|   stm32f765_767_777_bga176 IBIS Model
[IBIS ver]   4.2
[File name]  stm32f765_767_777_bga176.ibs
[File Rev]   1.0
[Date]   24-06-2015
[Source] Data Created at STMicroelectronics
[Notes]   File originated from ELDO simulations.
[Disclaimer]  This information is for modeling purpose only and is
   not guaranted. The information is subject to change without
   notice.
[Copyright] Copyright 2016 STMicroelectronics Inc.
[Component] stm32f765_767_777_bga176
[Manufacturer] STMicroelectronics
[Package]
| variable   typ   min   max
R_pkg   0.0   NA   NA
L_pkg   0.0H   NA   NA
C_pkg   0.0F   NA   NA
[Pin]   signal_name   model_name   R_pin   L_pin   C_pin
A1 PE3 io8p_arsudq_ft
A10 PB3 io8p_arsudq_ft
A11 PD7 io8p_arsudq_ft
A12 PC12 io8p_arsudq_ft
A13 PA15 io8p_arsudq_ft
A14 PA14 io8p_arsudq_ft
A15 PA13 io8p_arsudq_ft
A2 PE2 io8p_arsudq_ft
A3 PE1 io8p_arsudq_ft
A4 PE0 io8p_arsudq_ft
A5 PB8 io8p_arsudq_i2cin_ft
A6 PB5 io8p_ar3wsudq_ft
A7 PG14 io8p_arsudq_ft
A8 PG13 io8p_arsudq_ft
A9 PB4 io8p_arsudq_ft
B1 PE4 io8p_arsudq_ft
B10 PG10 io8p_arsudq_ft
B11 PD6 io8p_arsudq_ft
B12 PD0 io8p_arsudq_ft
B13 PC11 io8p_arsudq_ft
B14 PC10 io8p_arsudq_ft
B15 PA12 io8usb_lsfs_otg_ft
B2 PE5 io8p_arsudq_ft
B3 PE6 io8p_arsudq_ft
B4 PB9 io8p_arsudq_i2cin_ft
B5 PB7 io8p_arsudq_i2cin_ft
B6 PB6 io8p_arsudq_i2cin_ft
B7 PG15 io8p_arsudq_ft
B8 PG12 io8p_arsudq_ft
B9 PG11 io8p_arsudq_ft
C1 VBAT POWER
C10 PG9 io8p_arsudq_ft
C11 PD5 io8p_arsudq_ft
C12 PD1 io8p_arsudq_ft
C13 PI3 io8p_arsudq_ft
C14 PI2 io8p_arsudq_ft
C15 PA11 io8usb_lsfs_otg_ft
C2 PI7 io8p_arsudq_ft
C3 PI6 io8p_arsudq_ft
C4 PI5 io8p_arsudq_ft
C5 VDD POWER
C6 PDR_ON NC
C7 VDD POWER
C8 VDDSDMMC POWER
C9 VDD POWER
D1 PC13 io8p_arwsudq_ft_v33
D10 PD4 io8p_arsudq_ft
D11 PD3 io8p_arsudq_ft
D12 PD2 io8p_arsudq_ft
D13 PH15 io8p_arsudq_ft
D14 PI1 io8p_arsudq_ft
D15 PA10 io8usb_id_otg_ft
D2 PI8 io8p_arsudq_ft_v33
D3 PI9 io8p_arsudq_ft
D4 PI4 io8p_arsudq_ft
D5 VSS GND
D6 BOOT0 GND
D7 VSS GND
D8 VSS GND
D9 VSS GND
E1 PC14-OSC32_IN io8p_arwsudq_ft_v33
E12 PH13 io8p_arsudq_ft
E13 PH14 io8p_arsudq_ft
E14 PI0 io8p_arsudq_ft
E15 PA9 io8usb_vbus_otg_ft
E2 PF0 io8p_arsudq_i2cin_ft
E3 PI10 io8p_arsudq_ft
E4 PI11 io8p_arsudq_ft_v33
F1 PC15-OSC32_OUT io8p_arsudq_ft
F12 VSS GND
F13 VCAP_2 POWER
F14 PC9 io8p_arsudq_i2cin_ft
F15 PA8 io8p_arsudq_i2cin_ft
F2 VSS GND
F3 VDD POWER
F4 PH2 io8p_arsudq_ft
F6 VSS GND
F7 VSS GND
F8 VSS GND
F9 VSS GND
F10 VSS GND
G1 PH0-OSC_IN io8p_arsudq_ft
G12 VSS GND
G13 VDD POWER
G14 PC8 io8p_arsudq_ft
G15 PC7 io8p_arsudq_ft
G2 VSS GND
G3 VDD POWER
G4 PH3 io8p_arsudq_ft
G6 VSS GND
G7 VSS GND
G8 VSS GND
G9 VSS GND
G10 VSS GND
H1 PH1-OSC_OUT io8p_arsudq_ft
H12 VSS GND
H13 VDDUSB POWER
H14 PG8 io8p_arsudq_ft
H15 PC6 io8p_arsudq_ft
H2 PF2 io8p_arsudq_ft
H3 PF1 io8p_arsudq_i2cin_ft
H4 PH4 io8p_arsudq_i2cin_ft
H6 VSS GND
H7 VSS GND
H8 VSS GND
H9 VSS GND
H10 VSS GND
J1 NRST ioreset_ft_v33
J12 VDD POWER
J13 VDD POWER
J14 PG7 io8p_arsudq_ft
J15 PG6 io8p_arsudq_ft
J2 PF3 io8p_arwsudq_ft
J3 PF4 io8p_arwsudq_ft
J4 PH5 io8p_arsudq_i2cin_ft
J6 VSS GND
J7 VSS GND
J8 VSS GND
J9 VSS GND
J10 VSS GND
K1 PF7 io8p_arwsudq_ft
K12 PH12 io8p_arsudq_i2cin_ft
K13 PG5 io8p_arsudq_ft
K14 PG4 io8p_arsudq_ft
K15 PG3 io8p_arsudq_ft
K2 PF6 io8p_arwsudq_ft
K3 PF5 io8p_arwsudq_ft
K4 VDD POWER
K6 VSS GND
K7 VSS GND
K8 VSS GND
K9 VSS GND
K10 VSS GND
L1 PF10 io8p_arwsudq_ft
L12 PH11 io8p_arsudq_i2cin_ft
L13 PH10 io8p_arsudq_ft
L14 PD15 io8p_arsudq_ft
L15 PG2 io8p_arsudq_ft
L2 PF9 io8p_arwsudq_ft
L3 PF8 io8p_arwsudq_ft
L4 BYPASS_REG NC
M1 VSSA GND
M10 VCAP_1 POWER
M11 PH6 io8p_arsudq_ft
M12 PH8 io8p_arsudq_i2cin_ft
M13 PH9 io8p_arsudq_ft
M14 PD14 io8p_arsudq_ft
M15 PD13 io8p_arsudq_i2cin_ft
M2 PC0 io8p_ar3wsudq_ft
M3 PC1 io8p_ar3wsudq_ft_v33
M4 PC2 io8p_ar3wsudq_ft
M5 PC3 io8p_ar3wsudq_ft
M6 PB2 io8p_ar3wsudq_ft
M7 PG1 io8p_arsudq_ft
M8 VSS GND
M9 VSS GND
N1 VREF- GND
N10 VDD POWER
N11 PE13 io8p_arsudq_ft
N12 PH7 io8p_arsudq_i2cin_ft
N13 PD12 io8p_arsudq_i2cin_ft
N14 PD11 io8p_arsudq_ft
N15 PD10 io8p_arsudq_ft
N2 PA1 io8p_ar3wsudq_ft
N3 PA0-WKUP io8p_ar3wsudq_ft_v33
N4 PA4 io8p_ar3wsudq_ft
N5 PC4 io8p_ar3wsudq_ft
N6 PF13 io8p_arsudq_ft
N7 PG0 io8p_arsudq_ft
N8 VDD POWER
N9 VDD POWER
P1 VREF+ POWER
P10 PE11 io8p_arsudq_ft
P11 PE14 io8p_arsudq_ft
P12 PB12 io8usb_id_otg_ft
P13 PB13 io8usb_vbus_otg_ft
P14 PD9 io8p_arsudq_ft
P15 PD8 io8p_arsudq_ft
P2 PA2 io8p_ar3wsudq_ft_v33
P3 PA6 io8p_ar3wsudq_ft
P4 PA5 io8p_ar3wsudq_ft
P5 PC5 io8p_ar3wsudq_ft
P6 PF12 io8p_arsudq_ft
P7 PF15 io8p_arsudq_i2cin_ft
P8 PE8 io8p_arsudq_ft
P9 PE9 io8p_arsudq_ft
R1 VDDA POWER
R10 PE12 io8p_arsudq_ft
R11 PE15 io8p_ar3wsudq_ft
R12 PB10 io8p_arsudq_i2cin_ft
R13 PB11 io8p_arsudq_i2cin_ft
R14 PB14 io8usb_lsfs_otg_ft
R15 PB15 io8usb_lsfs_otg_ft
R2 PA3 io8p_ar3wsudq_ft
R3 PA7 io8p_ar3wsudq_ft
R4 PB1 io8p_ar3wsudq_ft
R5 PB0 io8p_ar3wsudq_ft
R6 PF11 io8p_arsudq_ft
R7 PF14 io8p_arsudq_i2cin_ft
R8 PE7 io8p_arsudq_ft
R9 PE10 io8p_arsudq_ft
[Diff Pin]   inv_pin   vdiff   tdelay_typ  tdelay_min  tdelay_max
C15   B15   200mV   NA   NA   NA
R14   R15   200mV   NA   NA   NA
[Model Selector] io8p_ar3wsudq_ft
io8p00_ar3wsudq_ft_pd_lv  "SPEED00 1P8V, PD=40kOhm"
io8p00_ar3wsudq_ft_pu_lv  "SPEED00 1P8V, PU=40kOhm"
io8p00_ar3wsudq_ft_lv  "SPEED00 1P8V"
io8p01_ar3wsudq_ft_pd_lv  "SPEED01 1P8V, PD=40kOhm"
io8p01_ar3wsudq_ft_pu_lv  "SPEED01 1P8V, PU=40kOhm"
io8p01_ar3wsudq_ft_lv  "SPEED01 1P8V"
io8p10_ar3wsudq_ft_pd_lv  "SPEED10 1P8V, PD=40kOhm"
io8p10_ar3wsudq_ft_pu_lv  "SPEED10 1P8V, PU=40kOhm"
io8p10_ar3wsudq_ft_lv  "SPEED10 1P8V"
io8p11_ar3wsudq_ft_pd_lv  "SPEED11 1P8V, PD=40kOhm"
io8p11_ar3wsudq_ft_pu_lv  "SPEED11 1P8V, PU=40kOhm"
io8p11_ar3wsudq_ft_lv  "SPEED11 1P8V"
io8p00_ar3wsudq_ft_pd  "SPEED00, PD=40kOhm"
io8p00_ar3wsudq_ft_pu  "SPEED00, PU=40kOhm"
io8p00_ar3wsudq_ft  "SPEED00"
io8p01_ar3wsudq_ft_pd  "SPEED01, PD=40kOhm"
io8p01_ar3wsudq_ft_pu  "SPEED01, PU=40kOhm"
io8p01_ar3wsudq_ft  "SPEED01"
io8p10_ar3wsudq_ft_pd  "SPEED10, PD=40kOhm"
io8p10_ar3wsudq_ft_pu  "SPEED10, PU=40kOhm"
io8p10_ar3wsudq_ft  "SPEED10"
io8p11_ar3wsudq_ft_pd  "SPEED11, PD=40kOhm"
io8p11_ar3wsudq_ft_pu  "SPEED11, PU=40kOhm"
io8p11_ar3wsudq_ft  "SPEED11"
[Model Selector] io8p_ar3wsudq_ft_v33
io8p00_ar3wsudq_ft_v33_pd_lv  "SPEED00 1P8V, PD=40kOhm"
io8p00_ar3wsudq_ft_v33_pu_lv  "SPEED00 1P8V, PU=40kOhm"
io8p00_ar3wsudq_ft_v33_lv  "SPEED00 1P8V"
io8p01_ar3wsudq_ft_v33_pd_lv  "SPEED01 1P8V, PD=40kOhm"
io8p01_ar3wsudq_ft_v33_pu_lv  "SPEED01 1P8V, PU=40kOhm"
io8p01_ar3wsudq_ft_v33_lv  "SPEED01 1P8V"
io8p10_ar3wsudq_ft_v33_pd_lv  "SPEED10 1P8V, PD=40kOhm"
io8p10_ar3wsudq_ft_v33_pu_lv  "SPEED10 1P8V, PU=40kOhm"
io8p10_ar3wsudq_ft_v33_lv  "SPEED10 1P8V"
io8p11_ar3wsudq_ft_v33_pd_lv  "SPEED11 1P8V, PD=40kOhm"
io8p11_ar3wsudq_ft_v33_pu_lv  "SPEED11 1P8V, PU=40kOhm"
io8p11_ar3wsudq_ft_v33_lv  "SPEED11 1P8V"
io8p00_ar3wsudq_ft_v33_pd  "SPEED00, PD=40kOhm"
io8p00_ar3wsudq_ft_v33_pu  "SPEED00, PU=40kOhm"
io8p00_ar3wsudq_ft_v33  "SPEED00"
io8p01_ar3wsudq_ft_v33_pd  "SPEED01, PD=40kOhm"
io8p01_ar3wsudq_ft_v33_pu  "SPEED01, PU=40kOhm"
io8p01_ar3wsudq_ft_v33  "SPEED01"
io8p10_ar3wsudq_ft_v33_pd  "SPEED10, PD=40kOhm"
io8p10_ar3wsudq_ft_v33_pu  "SPEED10, PU=40kOhm"
io8p10_ar3wsudq_ft_v33  "SPEED10"
io8p11_ar3wsudq_ft_v33_pd  "SPEED11, PD=40kOhm"
io8p11_ar3wsudq_ft_v33_pu  "SPEED11, PU=40kOhm"
io8p11_ar3wsudq_ft_v33  "SPEED11"
[Model Selector] io8p_arsudq_ft
io8p00_arsudq_ft_pd_lv  "SPEED00 1P8V, PD=40kOhm"
io8p00_arsudq_ft_pu_lv  "SPEED00 1P8V, PU=40kOhm"
io8p00_arsudq_ft_lv  "SPEED00 1P8V"
io8p01_arsudq_ft_pd_lv  "SPEED01 1P8V, PD=40kOhm"
io8p01_arsudq_ft_pu_lv  "SPEED01 1P8V, PU=40kOhm"
io8p01_arsudq_ft_lv  "SPEED01 1P8V"
io8p10_arsudq_ft_pd_lv  "SPEED10 1P8V, PD=40kOhm"
io8p10_arsudq_ft_pu_lv  "SPEED10 1P8V, PU=40kOhm"
io8p10_arsudq_ft_lv  "SPEED10 1P8V"
io8p11_arsudq_ft_pd_lv  "SPEED11 1P8V, PD=40kOhm"
io8p11_arsudq_ft_pu_lv  "SPEED11 1P8V, PU=40kOhm"
io8p11_arsudq_ft_lv  "SPEED11 1P8V"
io8p00_arsudq_ft_pd  "SPEED00, PD=40kOhm"
io8p00_arsudq_ft_pu  "SPEED00, PU=40kOhm"
io8p00_arsudq_ft  "SPEED00"
io8p01_arsudq_ft_pd  "SPEED01, PD=40kOhm"
io8p01_arsudq_ft_pu  "SPEED01, PU=40kOhm"
io8p01_arsudq_ft  "SPEED01"
io8p10_arsudq_ft_pd  "SPEED10, PD=40kOhm"
io8p10_arsudq_ft_pu  "SPEED10, PU=40kOhm"
io8p10_arsudq_ft  "SPEED10"
io8p11_arsudq_ft_pd  "SPEED11, PD=40kOhm"
io8p11_arsudq_ft_pu  "SPEED11, PU=40kOhm"
io8p11_arsudq_ft  "SPEED11"
[Model Selector] io8p_arsudq_i2cin_ft
io8p00_arsudq_i2cin_ft_pd_lv  "SPEED00 1P8V, PD=40kOhm"
io8p00_arsudq_i2cin_ft_pu_lv  "SPEED00 1P8V, PU=40kOhm"
io8p00_arsudq_i2cin_ft_lv  "SPEED00 1P8V"
io8p01_arsudq_i2cin_ft_pd_lv  "SPEED01 1P8V, PD=40kOhm"
io8p01_arsudq_i2cin_ft_pu_lv  "SPEED01 1P8V, PU=40kOhm"
io8p01_arsudq_i2cin_ft_lv  "SPEED01 1P8V"
io8p10_arsudq_i2cin_ft_pd_lv  "SPEED10 1P8V, PD=40kOhm"
io8p10_arsudq_i2cin_ft_pu_lv  "SPEED10 1P8V, PU=40kOhm"
io8p10_arsudq_i2cin_ft_lv  "SPEED10 1P8V"
io8p11_arsudq_i2cin_ft_pd_lv  "SPEED11 1P8V, PD=40kOhm"
io8p11_arsudq_i2cin_ft_pu_lv  "SPEED11 1P8V, PU=40kOhm"
io8p11_arsudq_i2cin_ft_lv  "SPEED11 1P8V"
io8p00_arsudq_i2cin_ft_pd  "SPEED00, PD=40kOhm"
io8p00_arsudq_i2cin_ft_pu  "SPEED00, PU=40kOhm"
io8p00_arsudq_i2cin_ft  "SPEED00"
io8p01_arsudq_i2cin_ft_pd  "SPEED01, PD=40kOhm"
io8p01_arsudq_i2cin_ft_pu  "SPEED01, PU=40kOhm"
io8p01_arsudq_i2cin_ft  "SPEED01"
io8p10_arsudq_i2cin_ft_pd  "SPEED10, PD=40kOhm"
io8p10_arsudq_i2cin_ft_pu  "SPEED10, PU=40kOhm"
io8p10_arsudq_i2cin_ft  "SPEED10"
io8p11_arsudq_i2cin_ft_pd  "SPEED11, PD=40kOhm"
io8p11_arsudq_i2cin_ft_pu  "SPEED11, PU=40kOhm"
io8p11_arsudq_i2cin_ft  "SPEED11"
[Model Selector] io8p_arwsudq_ft_v33
io8p00_arwsudq_ft_v33_pd_lv  "SPEED00 1P8V, PD=40kOhm"
io8p00_arwsudq_ft_v33_pu_lv  "SPEED00 1P8V, PU=40kOhm"
io8p00_arwsudq_ft_v33_lv  "SPEED00 1P8V"
io8p01_arwsudq_ft_v33_pd_lv  "SPEED01 1P8V, PD=40kOhm"
io8p01_arwsudq_ft_v33_pu_lv  "SPEED01 1P8V, PU=40kOhm"
io8p01_arwsudq_ft_v33_lv  "SPEED01 1P8V"
io8p10_arwsudq_ft_v33_pd_lv  "SPEED10 1P8V, PD=40kOhm"
io8p10_arwsudq_ft_v33_pu_lv  "SPEED10 1P8V, PU=40kOhm"
io8p10_arwsudq_ft_v33_lv  "SPEED10 1P8V"
io8p11_arwsudq_ft_v33_pd_lv  "SPEED11 1P8V, PD=40kOhm"
io8p11_arwsudq_ft_v33_pu_lv  "SPEED11 1P8V, PU=40kOhm"
io8p11_arwsudq_ft_v33_lv  "SPEED11 1P8V"
io8p00_arwsudq_ft_v33_pd  "SPEED00, PD=40kOhm"
io8p00_arwsudq_ft_v33_pu  "SPEED00, PU=40kOhm"
io8p00_arwsudq_ft_v33  "SPEED00"
io8p01_arwsudq_ft_v33_pd  "SPEED01, PD=40kOhm"
io8p01_arwsudq_ft_v33_pu  "SPEED01, PU=40kOhm"
io8p01_arwsudq_ft_v33  "SPEED01"
io8p10_arwsudq_ft_v33_pd  "SPEED10, PD=40kOhm"
io8p10_arwsudq_ft_v33_pu  "SPEED10, PU=40kOhm"
io8p10_arwsudq_ft_v33  "SPEED10"
io8p11_arwsudq_ft_v33_pd  "SPEED11, PD=40kOhm"
io8p11_arwsudq_ft_v33_pu  "SPEED11, PU=40kOhm"
io8p11_arwsudq_ft_v33  "SPEED11"
[Model Selector] io8usb_id_otg_ft
io8p00_id_otg_ft_pd_lv  "SPEED00 1P8V, PD=14kOhm"
io8p00_id_otg_ft_pu_lv  "SPEED00 1P8V, PU=14kOhm"
io8p00_id_otg_ft_lv  "SPEED00 1P8V"
io8p01_id_otg_ft_pd_lv  "SPEED01 1P8V, PD=14kOhm"
io8p01_id_otg_ft_pu_lv  "SPEED01 1P8V, PU=14kOhm"
io8p01_id_otg_ft_lv  "SPEED01 1P8V"
io8p10_id_otg_ft_pd_lv  "SPEED10 1P8V, PD=14kOhm"
io8p10_id_otg_ft_pu_lv  "SPEED10 1P8V, PU=14kOhm"
io8p10_id_otg_ft_lv  "SPEED10 1P8V"
io8p11_id_otg_ft_pd_lv  "SPEED11 1P8V, PD=14kOhm"
io8p11_id_otg_ft_pu_lv  "SPEED11 1P8V, PU=14kOhm"
io8p11_id_otg_ft_lv  "SPEED11 1P8V"
io8p00_id_otg_ft_pd  "SPEED00, PD=14kOhm"
io8p00_id_otg_ft_pu  "SPEED00, PU=14kOhm"
io8p00_id_otg_ft  "SPEED00"
io8p01_id_otg_ft_pd  "SPEED01, PD=14kOhm"
io8p01_id_otg_ft_pu  "SPEED01, PU=14kOhm"
io8p01_id_otg_ft  "SPEED01"
io8p10_id_otg_ft_pd  "SPEED10, PD=14kOhm"
io8p10_id_otg_ft_pu  "SPEED10, PU=14kOhm"
io8p10_id_otg_ft  "SPEED10"
io8p11_id_otg_ft_pd  "SPEED11, PD=14kOhm"
io8p11_id_otg_ft_pu  "SPEED11, PU=14kOhm"
io8p11_id_otg_ft  "SPEED11"
[Model Selector] io8usb_lsfs_otg_ft
io8usb_ls_otg_ft_dpdn_pd  "LS USB DP/DN IO + PD=20kOhm"
io8usb_ls_otg_ft_dpdn_pupu2  "LS USB DP/DN IO + PU/PU2=2.2kOhm"
io8usb_ls_otg_ft_dpdn_pu2  "LS USB DP/DN IO + PU2=1.2kOhm"
io8usb_ls_otg_ft_dpdn_pu  "LS USB DP/DN IO + PU=1.2kOhm"
io8usb_ls_otg_ft_dpdn  "LS USB DP/DN IO"
io8usb_fs_otg_ft_dpdn_pd  "HS USB DP/DN IO + PD=20kOhm"
io8usb_fs_otg_ft_dpdn_pupu2  "HS USB DP/DN IO + PU/PU2=2.2kOhm"
io8usb_fs_otg_ft_dpdn_pu2  "HS USB DP/DN IO + PU2=1.2kOhm"
io8usb_fs_otg_ft_dpdn_pu  "HS USB DP/DN IO + PU=1.2kOhm"
io8usb_fs_otg_ft_dpdn  "HS USB DP/DN IO"
io8p00_lsfs_otg_ft_pd_lv  "SPEED00 1P8V, PD=40kOhm"
io8p00_lsfs_otg_ft_pu_lv  "SPEED00 1P8V, PU=40kOhm"
io8p00_lsfs_otg_ft_lv  "SPEED00 1P8V"
io8p01_lsfs_otg_ft_pd_lv  "SPEED01 1P8V, PD=40kOhm"
io8p01_lsfs_otg_ft_pu_lv  "SPEED01 1P8V, PU=40kOhm"
io8p01_lsfs_otg_ft_lv  "SPEED01 1P8V"
io8p10_lsfs_otg_ft_pd_lv  "SPEED10 1P8V, PD=40kOhm"
io8p10_lsfs_otg_ft_pu_lv  "SPEED10 1P8V, PU=40kOhm"
io8p10_lsfs_otg_ft_lv  "SPEED10 1P8V"
io8p11_lsfs_otg_ft_pd_lv  "SPEED11 1P8V, PD=40kOhm"
io8p11_lsfs_otg_ft_pu_lv  "SPEED11 1P8V, PU=40kOhm"
io8p11_lsfs_otg_ft_lv  "SPEED11 1P8V"
io8p00_lsfs_otg_ft_pd  "SPEED00, PD=40kOhm"
io8p00_lsfs_otg_ft_pu  "SPEED00, PU=40kOhm"
io8p00_lsfs_otg_ft  "SPEED00"
io8p01_lsfs_otg_ft_pd  "SPEED01, PD=40kOhm"
io8p01_lsfs_otg_ft_pu  "SPEED01, PU=40kOhm"
io8p01_lsfs_otg_ft  "SPEED01"
io8p10_lsfs_otg_ft_pd  "SPEED10, PD=40kOhm"
io8p10_lsfs_otg_ft_pu  "SPEED10, PU=40kOhm"
io8p10_lsfs_otg_ft  "SPEED10"
io8p11_lsfs_otg_ft_pd  "SPEED11, PD=40kOhm"
io8p11_lsfs_otg_ft_pu  "SPEED11, PU=40kOhm"
io8p11_lsfs_otg_ft  "SPEED11"
[Model Selector] io8usb_vbus_otg_ft
io8psenb_vbus_otg_ft  "VBUS PULSE, SENSE VB"
io8psenab_vbus_otg_ft  "VBUS PULSE, SENSE VA and VB"
io8psena_vbus_otg_ft  "VBUS PULSE, SENSE VA"
io8psen_vbus_otg_ft  "VBUS PULSE"
io8p00_vbus_otg_ft_pd_lv  "SPEED00 1P8V, PD=40kOhm"
io8p00_vbus_otg_ft_pu_lv  "SPEED00 1P8V, PU=40kOhm"
io8p00_vbus_otg_ft_lv  "SPEED00 1P8V"
io8p01_vbus_otg_ft_pd_lv  "SPEED01 1P8V, PD=40kOhm"
io8p01_vbus_otg_ft_pu_lv  "SPEED01 1P8V, PU=40kOhm"
io8p01_vbus_otg_ft_lv  "SPEED01 1P8V"
io8p10_vbus_otg_ft_pd_lv  "SPEED10 1P8V, PD=40kOhm"
io8p10_vbus_otg_ft_pu_lv  "SPEED10 1P8V, PU=40kOhm"
io8p10_vbus_otg_ft_lv  "SPEED10 1P8V"
io8p11_vbus_otg_ft_pd_lv  "SPEED11 1P8V, PD=40kOhm"
io8p11_vbus_otg_ft_pu_lv  "SPEED11 1P8V, PU=40kOhm"
io8p11_vbus_otg_ft_lv  "SPEED11 1P8V"
io8p00_vbus_otg_ft_pd  "SPEED00, PD=40kOhm"
io8p00_vbus_otg_ft_pu  "SPEED00, PU=40kOhm"
io8p00_vbus_otg_ft  "SPEED00"
io8p01_vbus_otg_ft_pd  "SPEED01, PD=40kOhm"
io8p01_vbus_otg_ft_pu  "SPEED01, PU=40kOhm"
io8p01_vbus_otg_ft  "SPEED01"
io8p10_vbus_otg_ft_pd  "SPEED10, PD=40kOhm"
io8p10_vbus_otg_ft_pu  "SPEED10, PU=40kOhm"
io8p10_vbus_otg_ft  "SPEED10"
io8p11_vbus_otg_ft_pd  "SPEED11, PD=40kOhm"
io8p11_vbus_otg_ft_pu  "SPEED11, PU=40kOhm"
io8p11_vbus_otg_ft  "SPEED11"
[Model Selector] ioreset_ft_v33
ioreset_ft_v33_pu_lv  "ioreset 1P8V + PU=40kOhm"
ioreset_ft_v33_nopu_lv  "ioreset 1P8V"
ioreset_ft_v33_pu  "ioreset + PU=40kOhm"
ioreset_ft_v33_nopu  "ioreset"
[Model Selector] io8p_arwsudq_ft
io8p00_arwsudq_ft_pd_lv  "SPEED00 1P8V, PD=40kOhm"
io8p00_arwsudq_ft_pu_lv  "SPEED00 1P8V, PU=40kOhm"
io8p00_arwsudq_ft_lv  "SPEED00 1P8V"
io8p01_arwsudq_ft_pd_lv  "SPEED01 1P8V, PD=40kOhm"
io8p01_arwsudq_ft_pu_lv  "SPEED01 1P8V, PU=40kOhm"
io8p01_arwsudq_ft_lv  "SPEED01 1P8V"
io8p10_arwsudq_ft_pd_lv  "SPEED10 1P8V, PD=40kOhm"
io8p10_arwsudq_ft_pu_lv  "SPEED10 1P8V, PU=40kOhm"
io8p10_arwsudq_ft_lv  "SPEED10 1P8V"
io8p11_arwsudq_ft_pd_lv  "SPEED11 1P8V, PD=40kOhm"
io8p11_arwsudq_ft_pu_lv  "SPEED11 1P8V, PU=40kOhm"
io8p11_arwsudq_ft_lv  "SPEED11 1P8V"
io8p00_arwsudq_ft_pd  "SPEED00, PD=40kOhm"
io8p00_arwsudq_ft_pu  "SPEED00, PU=40kOhm"
io8p00_arwsudq_ft  "SPEED00"
io8p01_arwsudq_ft_pd  "SPEED01, PD=40kOhm"
io8p01_arwsudq_ft_pu  "SPEED01, PU=40kOhm"
io8p01_arwsudq_ft  "SPEED01"
io8p10_arwsudq_ft_pd  "SPEED10, PD=40kOhm"
io8p10_arwsudq_ft_pu  "SPEED10, PU=40kOhm"
io8p10_arwsudq_ft  "SPEED10"
io8p11_arwsudq_ft_pd  "SPEED11, PD=40kOhm"
io8p11_arwsudq_ft_pu  "SPEED11, PU=40kOhm"
io8p11_arwsudq_ft  "SPEED11"
[Model Selector] io8p_arsudq_ft_v33
io8p00_arsudq_ft_v33_pd_lv  "SPEED00 1P8V, PD=40kOhm"
io8p00_arsudq_ft_v33_pu_lv  "SPEED00 1P8V, PU=40kOhm"
io8p00_arsudq_ft_v33_lv  "SPEED00 1P8V"
io8p01_arsudq_ft_v33_pd_lv  "SPEED01 1P8V, PD=40kOhm"
io8p01_arsudq_ft_v33_pu_lv  "SPEED01 1P8V, PU=40kOhm"
io8p01_arsudq_ft_v33_lv  "SPEED01 1P8V"
io8p10_arsudq_ft_v33_pd_lv  "SPEED10 1P8V, PD=40kOhm"
io8p10_arsudq_ft_v33_pu_lv  "SPEED10 1P8V, PU=40kOhm"
io8p10_arsudq_ft_v33_lv  "SPEED10 1P8V"
io8p11_arsudq_ft_v33_pd_lv  "SPEED11 1P8V, PD=40kOhm"
io8p11_arsudq_ft_v33_pu_lv  "SPEED11 1P8V, PU=40kOhm"
io8p11_arsudq_ft_v33_lv  "SPEED11 1P8V"
io8p00_arsudq_ft_v33_pd  "SPEED00, PD=40kOhm"
io8p00_arsudq_ft_v33_pu  "SPEED00, PU=40kOhm"
io8p00_arsudq_ft_v33  "SPEED00"
io8p01_arsudq_ft_v33_pd  "SPEED01, PD=40kOhm"
io8p01_arsudq_ft_v33_pu  "SPEED01, PU=40kOhm"
io8p01_arsudq_ft_v33  "SPEED01"
io8p10_arsudq_ft_v33_pd  "SPEED10, PD=40kOhm"
io8p10_arsudq_ft_v33_pu  "SPEED10, PU=40kOhm"
io8p10_arsudq_ft_v33  "SPEED10"
io8p11_arsudq_ft_v33_pd  "SPEED11, PD=40kOhm"
io8p11_arsudq_ft_v33_pu  "SPEED11, PU=40kOhm"
io8p11_arsudq_ft_v33  "SPEED11"
| Models and submodels in the file (258): io8p00_ar3wsudq_ft_pd_lv (I/O), io8p00_ar3wsudq_ft_pu_lv (I/O), io8p00_ar3wsudq_ft_lv (I/O), io8p01_ar3wsudq_ft_pd_lv (I/O), io8p01_ar3wsudq_ft_pu_lv (I/O), io8p01_ar3wsudq_ft_lv (I/O), io8p10_ar3wsudq_ft_pd_lv (I/O), io8p10_ar3wsudq_ft_pu_lv (I/O), io8p10_ar3wsudq_ft_lv (I/O), io8p11_ar3wsudq_ft_pd_lv (I/O), io8p11_ar3wsudq_ft_pu_lv (I/O), io8p11_ar3wsudq_ft_lv (I/O), io8p00_ar3wsudq_ft_pd (I/O), io8p00_ar3wsudq_ft_pu (I/O), io8p00_ar3wsudq_ft (I/O), io8p01_ar3wsudq_ft_pd (I/O), io8p01_ar3wsudq_ft_pu (I/O), io8p01_ar3wsudq_ft (I/O), io8p10_ar3wsudq_ft_pd (I/O), io8p10_ar3wsudq_ft_pu (I/O), io8p10_ar3wsudq_ft (I/O), io8p11_ar3wsudq_ft_pd (I/O), io8p11_ar3wsudq_ft_pu (I/O), io8p11_ar3wsudq_ft (I/O), io8p00_ar3wsudq_ft_v33_pd_lv (I/O), io8p00_ar3wsudq_ft_v33_pu_lv (I/O), io8p00_ar3wsudq_ft_v33_lv (I/O), io8p01_ar3wsudq_ft_v33_pd_lv (I/O), io8p01_ar3wsudq_ft_v33_pu_lv (I/O), io8p01_ar3wsudq_ft_v33_lv (I/O), io8p10_ar3wsudq_ft_v33_pd_lv (I/O), io8p10_ar3wsudq_ft_v33_pu_lv (I/O), io8p10_ar3wsudq_ft_v33_lv (I/O), io8p11_ar3wsudq_ft_v33_pd_lv (I/O), io8p11_ar3wsudq_ft_v33_pu_lv (I/O), io8p11_ar3wsudq_ft_v33_lv (I/O), io8p00_ar3wsudq_ft_v33_pd (I/O), io8p00_ar3wsudq_ft_v33_pu (I/O), io8p00_ar3wsudq_ft_v33 (I/O), io8p01_ar3wsudq_ft_v33_pd (I/O), io8p01_ar3wsudq_ft_v33_pu (I/O), io8p01_ar3wsudq_ft_v33 (I/O), io8p10_ar3wsudq_ft_v33_pd (I/O), io8p10_ar3wsudq_ft_v33_pu (I/O), io8p10_ar3wsudq_ft_v33 (I/O), io8p11_ar3wsudq_ft_v33_pd (I/O), io8p11_ar3wsudq_ft_v33_pu (I/O), io8p11_ar3wsudq_ft_v33 (I/O), io8p00_arsudq_ft_pd_lv (I/O), io8p00_arsudq_ft_pu_lv (I/O), io8p00_arsudq_ft_lv (I/O), io8p01_arsudq_ft_pd_lv (I/O), io8p01_arsudq_ft_pu_lv (I/O), io8p01_arsudq_ft_lv (I/O), io8p10_arsudq_ft_pd_lv (I/O), io8p10_arsudq_ft_pu_lv (I/O), io8p10_arsudq_ft_lv (I/O), io8p11_arsudq_ft_pd_lv (I/O), io8p11_arsudq_ft_pu_lv (I/O), io8p11_arsudq_ft_lv (I/O), io8p00_arsudq_ft_pd (I/O), io8p00_arsudq_ft_pu (I/O), io8p00_arsudq_ft (I/O), io8p01_arsudq_ft_pd (I/O), io8p01_arsudq_ft_pu (I/O), io8p01_arsudq_ft (I/O), io8p10_arsudq_ft_pd (I/O), io8p10_arsudq_ft_pu (I/O), io8p10_arsudq_ft (I/O), io8p11_arsudq_ft_pd (I/O), io8p11_arsudq_ft_pu (I/O), io8p11_arsudq_ft (I/O), io8p00_arsudq_i2cin_ft_pd_lv (I/O), io8p00_arsudq_i2cin_ft_pu_lv (I/O), io8p00_arsudq_i2cin_ft_lv (I/O), io8p01_arsudq_i2cin_ft_pd_lv (I/O), io8p01_arsudq_i2cin_ft_pu_lv (I/O), io8p01_arsudq_i2cin_ft_lv (I/O), io8p10_arsudq_i2cin_ft_pd_lv (I/O), io8p10_arsudq_i2cin_ft_pu_lv (I/O)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
